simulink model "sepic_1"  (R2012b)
settings: Solver=ode45  StartTime=0.0  StopTime=10.0  RelTol=1e-3
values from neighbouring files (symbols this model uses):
  C1 = 200e-6    (= 0.0002)    [Cuk1.m]    (also in sepic1.m = 0.0001; sepic2.m = 0.0001; feder_masse_1.m = [1 0 0 0]; feder_masse_13.m = [1 0 0 0])
  C2 = C1    (= 0.0002)    [Cuk1.m]    (also in sepic1.m = 0.0001; sepic2.m = 0.0001; feder_masse_1.m = [0 0 1 0]; feder_masse_13.m = [0 0 1 0])
  f0 = 0.2e5    (= 20000)    [boost_up1.m]    (also in buck_boost1.m; buck_boost2.m; buck_down1.m; buck_down2.m)
  L1 = 0.0001    [Cuk1.m]    (also in sepic1.m = 5e-05; sepic2.m = 5e-05)
  L2 = L1    (= 0.0001)    [Cuk1.m]    (also in sepic1.m = 5e-05; sepic2.m = 5e-05)
  R = 5    [boost_up1.m]    (also in buck_boost1.m; buck_boost2.m; buck_down1.m = 2*Rmax,; buck_down2.m = 0.1*Rmax,)
  T = 1/f0    (= 5e-05)    [boost_up1.m]    (also in buck_boost1.m; buck_boost2.m; buck_down1.m; buck_down2.m)
  T1 = T-T2    (= 2.5e-05)    [buck_boost1.m]    (also in buck_boost2.m = 1e-05; sepic1.m = T-T2; sepic2.m = T-T2; unwucht_4.m = 500)
  Ui = 5    [boost_up1.m]    (also in buck_boost1.m; buck_boost2.m; buck_down1.m; buck_down2.m)

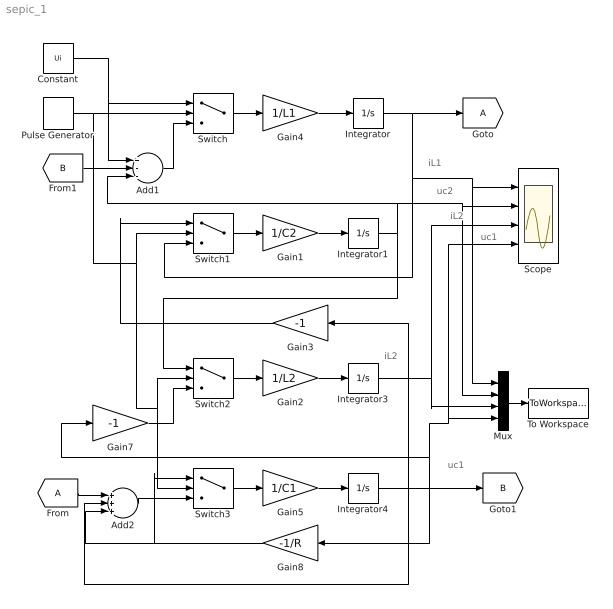
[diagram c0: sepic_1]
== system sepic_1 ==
  note: uc1
  note: iL2
  note: uc1
  note: iL2
  note: uc2
  note: iL1
  Add1 : Sum  Inputs=+--
  Add2 : Sum  Inputs=+++
  Constant : Constant  Value=Ui
  From : From
  Gain1 : Gain  Gain=1/C2
  Gain2 : Gain  Gain=1/L2
  Gain3 : Gain  Gain=-1
  Gain4 : Gain  Gain=1/L1
  Gain5 : Gain  Gain=1/C1
  Gain7 : Gain  Gain=-1
  Gain8 : Gain  Gain=-1/R
  Integrator{,1,3..4} (4 alike) : Integrator
  Mux : Mux
  Pulse Generator : DiscretePulseGenerator  PulseType=Time based  Period=1/f0  PulseWidth=T1*100/T
  Scope : Scope  NumInputPorts=4
  Switch{,1..3} (4 alike) : Switch  Criteria=u2 > Threshold  Threshold=0.5  ZeroCross=off  SampleTime=0
  To Workspace : ToWorkspace  VariableName=y  SampleTime=-1  SaveFormat=Structure With Time
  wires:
  Constant/1 -> Add1/1, Switch/1
  Pulse Generator/1 -> Switch/2, Switch3/2, Switch2/2, Switch1/2
  Add1/1 -> Switch/3
  Switch/1 -> Gain4/1
  Gain4/1 -> Integrator/1
  Switch1/1 -> Gain1/1
  Gain1/1 -> Integrator1/1
  Integrator1/1 -> Switch2/1, Add1/3, Mux/2, Scope/2
  Switch2/1 -> Gain2/1
  Gain2/1 -> Integrator3/1
  Integrator/1 -> Mux/1, Scope/1, Switch1/3, [A]
  Gain7/1 -> Switch2/3
  Mux/1 -> To Workspace/1
  Switch3/1 -> Gain5/1
  Gain5/1 -> Integrator4/1
  Add2/1 -> Switch3/3
  From/1 -> Add2/1
  Integrator3/1 -> Add2/2, Gain3/1, Mux/3, Scope/3
  Integrator4/1 -> Gain7/1, Scope/4, Mux/4, Gain8/1, [B]
  Gain8/1 -> Add2/3, Switch3/1
  [B] -> Add1/2
  Gain3/1 -> Switch1/1
